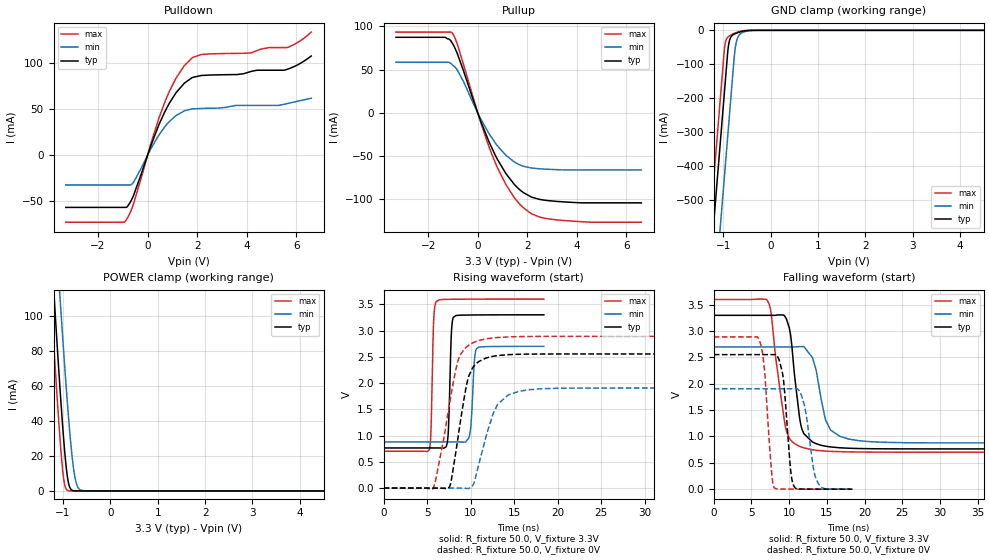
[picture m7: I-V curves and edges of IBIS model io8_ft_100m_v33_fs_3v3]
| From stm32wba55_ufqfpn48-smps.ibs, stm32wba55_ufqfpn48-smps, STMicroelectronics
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[Model]   io8_ft_100m_v33_fs_3v3
Model_type I/O
Polarity   Non-Inverting
Enable   Active-Low
| CAP_THRESHOLD on pad IOFT is "UDTCAPC" :
| Rising=30.0% of vddiom   Falling=70.0% of vddiom
| C_comp min and max val. don't necessarily correlate with the min and max pvt
| but are the smallest and greatest pad capacitance found.
| var   typ   min   max
C_comp   2.72385pF  2.64024pF  2.77561pF
|C_comp_pullup   1.81451pF  1.75565pF  1.84959pF
|C_comp_pulldown   909.34185fF  884.59080fF  926.01520fF
Vinl = 1.35V
Vinh = 1.8V
Vmeas = 1.65V   | Reference voltage for timing measurements
Cref  = 50.0pF   | Timing specification test load capacitance value
Rref  = 1.0MOhm   | Timing specification test load resistance value
Vref  = 1.815V   | Timing specification test load voltage
[Model Spec]
| TIME_THRESHOLD on pin ZIV33M is "CMOS" :
| Rising=50.0% of vddiom   Falling=50.0% of vddiom
Vinl 1.28450V 1.07650V 1.38450V
Vinh 1.79550V 1.49050V 1.94250V
| variable   typ   min   max
[Temperature Range] 25.0 140.0 -40.0
| variable   typ   min   max
[Voltage Range] 3.3V 2.7V 3.6V
| variable   typ   min   max
[POWER Clamp Reference] 3.3V 2.7V 3.6V
| variable   typ   min   max
[GND Clamp Reference] 0V 0V 0V
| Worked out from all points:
|   slope of the pulldown table from 0 to 0.495 V, typ, clamps not added: 14 ohm
|   slope of the pullup table from 0 to 0.495 V, typ, clamps not added: 13.8 ohm
|   GND clamp passes 1 mA (typ) near -0.51 V on its own axis
|   POWER clamp passes 1 mA (typ) near -0.83 V on its own axis
|   rising waveform, R_fixture 50.0, V_fixture 3.3V: 20-80 % time 262ps typ, 340ps min, 238ps max; typ from 0.764 V to 3.3 V
|   falling waveform, R_fixture 50.0, V_fixture 3.3V: 20-80 % time 1.18ns typ, 1.66ns min, 1.56ns max; typ from 3.3 V to 0.764 V
|   rising waveform, R_fixture 50.0, V_fixture 0V: 20-80 % time 1.51ns typ, 2.07ns min, 1.89ns max; typ from 0 V to 2.55 V
|   falling waveform, R_fixture 50.0, V_fixture 0V: 20-80 % time 833ps typ, 1.11ns min, 843ps max; typ from 2.55 V to 0 V
[POWER Clamp]
-3.3V     1.123A     1.139A     1.091A
-1.36V    189.2mA    238.8mA    158.1mA
-1.25V    139mA      190.3mA    108.1mA
-1.18V    107.9mA    159.9mA    77.22mA
-1.06V    57.23mA    109.3mA    28.68mA
-980mV    27.6mA     77.28mA    5.935mA
-900mV    6.895mA    47.74mA    242.8uA
-820mV    594.6uA    22.85mA    5.912uA
-760mV    69.41uA    9.714mA    358.6nA
-700mV    7.83uA     2.919mA    21.86nA
-630mV    611.5nA    529.9uA    954.5pA
6.6V      0A         0A         0A
[GND Clamp]
-3.3V     -4.134A    -4.382A    -4.006A
-1.59V    -1.227A    -1.475A    -1.099A
-1.25V    -648.9mA   -896.7mA   -520.9mA
-980mV    -189.9mA   -437.7mA   -61.92mA
-970mV    -172.9mA   -420.7mA   -48.45mA
-910mV    -70.86mA   -318.7mA   -21.03mA
-880mV    -37.23mA   -267.7mA   -17.31mA
-750mV    -9.908mA   -55.25mA   -7.768mA
-710mV    -7.626mA   -27.41mA   -5.608mA
-650mV    -4.885mA   -11.6mA    -3.058mA
-360mV    -31.22uA   -443.6uA   -1.188uA
6.6V      2.31nA     2.655uA    974.6pA
| variable   typ   min   max
[Pullup Reference] 3.3V 2.7V 3.6V
| variable   typ   min   max
[Pulldown Reference] 0V 0V 0V
[Pullup]
-3.3V     87.4mA     58.48mA    93.44mA
-1.32V    87.4mA     58.48mA    93.44mA
-1.01V    79.96mA    55.17mA    91.59mA
-840mV    69.65mA    50.07mA    80.67mA
-570mV    48.3mA     36.04mA    55.62mA
120mV     -9.566mA   -6.929mA   -11.25mA
710mV     -49.08mA   -34.92mA   -57.81mA
1.14V     -70.33mA   -49.14mA   -83.06mA
1.83V     -91.98mA   -61.62mA   -109.5mA
2.17V     -97.42mA   -63.75mA   -116.7mA
2.85V     -101.5mA   -65.23mA   -122.5mA
6.6V      -104mA     -65.97mA   -126.4mA
[Pulldown]
-3.3V     -56.7mA    -32.4mA    -72.73mA
-890mV    -56.7mA    -32.4mA    -71.32mA
-570mV    -43.94mA   -29.54mA   -52.99mA
120mV     9.474mA    6.407mA    11.48mA
700mV     47.33mA    30.97mA    57.88mA
1.14V     67.41mA    42.74mA    83.2mA
1.78V     83.75mA    50.04mA    105.1mA
2.17V     86.37mA    50.65mA    109.1mA
4.16V     90.65mA    53.91mA    110.8mA
4.9V      92.06mA    53.91mA    116.6mA
5.63V     93.04mA    55.89mA    116.6mA
6.6V      107.5mA    61.71mA    133.4mA
[Ramp]
dV/dt_r 1.53258V/1.50295ns 1.14345V/2.03095ns 1.73412V/1.84246ns
dV/dt_f 1.52157V/1.17988ns 1.09312V/1.53126ns 1.73923V/1.55395ns
R_load = 50.0
| Removed startup time: 0s 0s 0s  .
| Removed end time: 18.4ns.
[Rising Waveform]
R_fixture   = 50.0
V_fixture   = 3.3V
V_fixture_min = 2.7V
V_fixture_max = 3.6V
0s        764mV      878.1mV    701.3mV
5.25ns    764.1mV    878.1mV    742.1mV
5.45ns    764.1mV    878.1mV    1.178V
5.75ns    764.1mV    878.1mV    3.217V
6.05ns    764.1mV    878.1mV    3.554V
7.35ns    919.8mV    878.1mV    3.595V
8ns       3.251V     878.1mV    3.596V
9.85ns    3.296V     992.7mV    3.598V
10.65ns   3.297V     2.65V      3.599V
18.4ns    3.3V       2.7V       3.6V
| Removed startup time: 0s 0s 0s  .
| Removed end time: 58.4ns.
[Falling Waveform]
R_fixture   = 50.0
V_fixture   = 3.3V
V_fixture_min = 2.7V
V_fixture_max = 3.6V
0s        3.3V       2.7V       3.6V
7.15ns    3.3V       2.7V       3.57V
7.6ns     3.3V       2.7V       3.346V
9.3ns     3.303V     2.7V       1.365V
10ns      3.067V     2.7V       971.4mV
11.55ns   1.219V     2.706V     802.1mV
13.1ns    894.1mV    2.494V     747.6mV
15.5ns    801.7mV    1.12V      717.8mV
17.9ns    777.2mV    951.4mV    708mV
58.4ns    764.1mV    878.1mV    701.3mV
| Removed startup time: 0s 0s 0s  .
| Removed end time: 58.4ns.
[Rising Waveform]
R_fixture   = 50.0
V_fixture   = 0V
V_fixture_min = 0V
V_fixture_max = 0V
0s        20.88nV    574.1nV    33.14nV
5.65ns    5.621uV    585.7nV    -15.25mV
7.5ns     12.33mV    2.895uV    1.546V
8.7ns     1.144V     59.1uV     2.498V
9.7ns     2.09V      -7.751mV   2.712V
10.3ns    2.309V     68.6mV     2.771V
10.75ns   2.388V     339.1mV    2.802V
13.1ns    2.524V     1.598V     2.868V
15.5ns    2.548V     1.841V     2.885V
58.4ns    2.554V     1.906V     2.89V
| Removed startup time: 0s 0s 0s  .
| Removed end time: 18.4ns.
[Falling Waveform]
R_fixture   = 50.0
V_fixture   = 0V
V_fixture_min = 0V
V_fixture_max = 0V
0s        2.554V     1.906V     2.89V
6ns       2.554V     1.906V     2.841V
6.75ns    2.554V     1.906V     2.224V
7.65ns    2.554V     1.906V     363.1mV
8.05ns    2.554V     1.906V     20.42mV
9.2ns     2.12V      1.906V     2.083mV
10.6ns    65.13mV    1.906V     1.158mV
12.05ns   2.091mV    1.578V     814.8uV
13.95ns   1.02mV     85.22mV    517.4uV
18.4ns    292.7uV    1.262mV    146uV
